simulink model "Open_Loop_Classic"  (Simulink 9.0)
settings: Solver=ode45  StartTime=0.0  StopTime=40  RelTol=1e-3  EnableMultiTasking=on
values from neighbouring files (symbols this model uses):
  d2r = 1/r2d    (= 0.0174532925199)    [init.m]    (also in freq.m; frequ.m; init_lat.m; pl.m)
  r2d = 180/pi    (= 57.2957795131)    [init.m]    (also in freq.m; frequ.m; init_lat.m; pl.m)
undefined symbols (not defined in the file or in its folder): Av, Bv, Cv, Dv

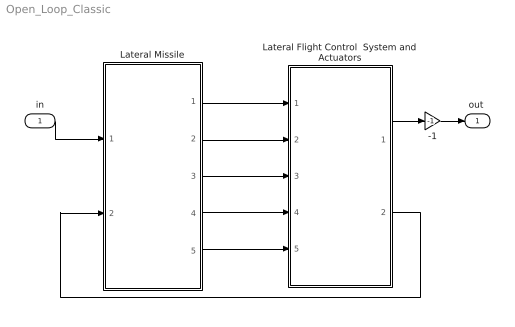
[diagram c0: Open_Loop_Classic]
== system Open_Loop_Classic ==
  in : Inport
  -1 : Gain  Gain=-1
  Lateral Flight Control  System and Actuators : Subsystem
  Lateral Missile : Subsystem
  "out " : Outport
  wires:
  Lateral Missile/1(p) -> Lateral Flight Control  System and Actuators/1(p)
  Lateral Missile/2(phi) -> Lateral Flight Control  System and Actuators/2(phi)
  Lateral Missile/3(r) -> Lateral Flight Control  System and Actuators/3(r)
  Lateral Missile/4(psi) -> Lateral Flight Control  System and Actuators/4(psi)
  Lateral Missile/5(Ny) -> Lateral Flight Control  System and Actuators/5(Nym)
  -1/1 -> "out "/1
  Lateral Flight Control  System and Actuators/1(d-ailer) -> -1/1
  in/1 -> Lateral Missile/1(dail)
  Lateral Flight Control  System and Actuators/2(d-ruddr) -> Lateral Missile/2(drud)

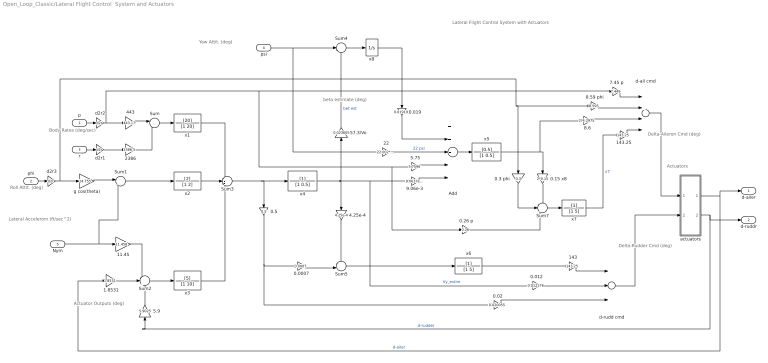
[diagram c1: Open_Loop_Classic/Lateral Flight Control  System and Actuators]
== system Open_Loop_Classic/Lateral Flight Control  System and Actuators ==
  note: Body Rates (deg/sec)
  note: Delta-Rudder Cmd (deg)
  note: Delta-Aileron Cmd (deg)
  note: Lateral Accelerom (ft/sec^2)
  note: Actuator Outputs (deg)
  note: Roll Attit. (deg)
  note: Yaw Attit. (deg)
  note: beta estimate (deg)
  note: Actuators
  note: Lateral Flight Control System with Actuators
  p : Inport
  phi : Inport  Port=2
  r : Inport  Port=3
  psi : Inport  Port=4
  Nym : Inport  Port=5
  0.0007 : Gain  Gain=0.0007
  0.012 : Gain  Gain=0.012176
  0.019 : Gain  Gain=0.019199
  0.02 : Gain  Gain=0.020055
  0.15 x8 : Gain  Gain=2*0.15
  0.26 p : Gain  Gain=0.26
  0.3 phi : Gain  Gain=0.3
  0.5 : Gain  Gain=0.5
  1.8531 : Gain  Gain=1.8531
  11.45 : Gain  Gain=11.458
  143 : Gain  Gain=143.25
  143.25 : Gain  Gain=143.25
  22 : Gain  Gain=22.002*d2r
  2386 : Gain  Gain=2386.5
  4.25e-4 : Gain  Gain=4.25e-4
  443 : Gain  Gain=443.17
  5.75 : Gain  Gain=5.7596
  5.9 : Gain  Gain=5.9025
  57.3/Vo : Gain  Gain=0.023605
  7.45 p : Gain  Gain=7.449
  8.59 phi : Gain  Gain=8.595
  8.6 : Gain  Gain=2*4.2975
  "9.06e-3 " : Gain  Gain=9.0637e-3
  Add : Sum  Inputs=++---
  Sum : Sum  Inputs=|-+
  Sum1 : Sum  Inputs=|++
  Sum2 : Sum  Inputs=-++
  Sum3 : Sum  Inputs=-++
  Sum4 : Sum  Inputs=+--
  Sum5 : Sum  Inputs=--|
  Sum7 : Sum  Inputs=-++
  actuators : Subsystem
  d-ail cmd : Sum  Inputs=++-+
  d-rudd cmd : Sum  Inputs=+--
  d2r1 : Gain  Gain=d2r
  d2r2 : Gain  Gain=d2r
  d2r3 : Gain  Gain=d2r
  g cos(theta) : Gain  Gain=24.755
  x1 : TransferFcn  Numerator=[20]  Denominator=[1 20]
  x2 : TransferFcn  Numerator=[2]  Denominator=[1 2]
  x3 : TransferFcn  Numerator=[5]  Denominator=[1 10]
  x4 : TransferFcn  Denominator=[1 0.5]
  x5 : TransferFcn  Numerator=[0.5]  Denominator=[1 0.5]
  x6 : TransferFcn  Denominator=[1 5]
  x7 : TransferFcn  Denominator=[1 5]
  x8 : Integrator
  d-ailer : Outport
  d-ruddr : Outport  Port=2
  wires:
  0.5/1 -> 0.02/1, 0.0007/1
  d-rudd cmd/1 -> actuators/2(dr)
  0.02/1 -> d-rudd cmd/3
  0.012/1 -> d-rudd cmd/2
  x6/1 -> 143/1
  143/1 -> d-rudd cmd/1
  d-ail cmd/1 -> actuators/1(da)
  7.45 p/1 -> d-ail cmd/1
  8.59 phi/1 -> d-ail cmd/2
  143.25/1 -> d-ail cmd/4
  x7/1 -> 143.25/1  "x7"
  8.6/1 -> d-ail cmd/3
  0.3 phi/1 -> Sum7/2
  0.26 p/1 -> Sum7/3
  0.15 x8/1 -> Sum7/1
  Sum7/1 -> x7/1
  x5/1 -> 8.6/1, 0.15 x8/1
  5.75/1 -> Add/4
  22/1 -> Add/3  "22 psi"
  0.019/1 -> Add/2
  x8/1 -> 0.019/1
  Add/1 -> x5/1
  "9.06e-3 "/1 -> Add/5
  Sum5/1 -> x6/1
  0.0007/1 -> Sum5/2
  4.25e-4/1 -> Sum5/1
  Nym/1 -> Sum1/2, 11.45/1
  Sum4/1 -> x8/1
  57.3/Vo/1 -> Sum4/3  "bet est"
  x4/1 -> 0.012/1, "9.06e-3 "/1, 4.25e-4/1, 57.3/Vo/1  "Vy_estim"
  psi/1 -> Sum4/2, 22/1
  Sum3/1 -> 0.5/1, x4/1
  x3/1 -> Sum3/3
  x2/1 -> Sum3/2
  x1/1 -> Sum3/1
  Sum2/1 -> x3/1
  5.9/1 -> Sum2/3
  1.8531/1 -> Sum2/2
  11.45/1 -> Sum2/1
  phi/1 -> d2r3/1
  g cos(theta)/1 -> Sum1/1
  Sum1/1 -> x2/1
  2386/1 -> Sum/2
  r/1 -> d2r1/1
  p/1 -> d2r2/1
  443/1 -> Sum/1
  Sum/1 -> x1/1
  actuators/1("da ") -> d-ailer/1, 1.8531/1  "d-ailer"
  actuators/2("dr ") -> d-ruddr/1, 5.9/1  "d-rudder"
  d2r3/1 -> 8.59 phi/1, 0.3 phi/1, g cos(theta)/1
  d2r2/1 -> 7.45 p/1, 0.26 p/1, 5.75/1, 443/1
  d2r1/1 -> 2386/1

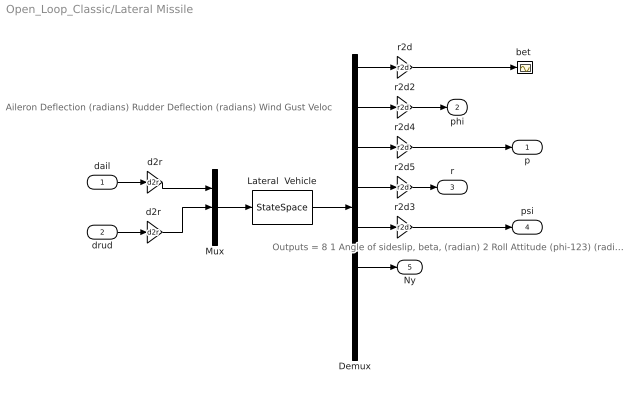
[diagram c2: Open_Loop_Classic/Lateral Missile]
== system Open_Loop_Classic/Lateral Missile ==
  note: Aileron Deflection (radians) Rudder Deflection (radians) Wind Gust Veloc
  note: Outputs = 8 1 Angle of sideslip, beta, (radian) 2 Roll Attitude (phi-123) (radians) 3 Roll Rate (p-body) (rad/sec) 4 Yaw Rate (r-body) (rad/sec) 5 Yaw Attitude (psi-123) (radians) 6 Y-Acceleromet, (ft/sec^2) Translation 7 Cross Range Velocity (Vcr) (ft/sec) 8 Beta Sensed at Vane # 1 (radian)
  dail : Inport
  drud : Inport  Port=2
  Demux : Demux  Outputs=8
  Lateral  Vehicle : StateSpace  A=Av  B=Bv  C=Cv  D=Dv  InitialCondition=0
  Mux : Mux  Inputs=3
  "bet " : Scope
  d2r : Gain  Gain=d2r
  "d2r " : Gain  Gain=d2r
  r2d{,2..5} (5 alike) : Gain  Gain=r2d
  p : Outport
  phi : Outport  Port=2
  r : Outport  Port=3
  psi : Outport  Port=4
  Ny : Outport  Port=5
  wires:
  Mux/1 -> Lateral  Vehicle/1
  Lateral  Vehicle/1 -> Demux/1
  dail/1 -> d2r/1
  drud/1 -> "d2r "/1
  r2d/1 -> "bet "/1
  Demux/1 -> r2d/1
  Demux/2 -> r2d2/1
  Demux/3 -> r2d4/1
  Demux/4 -> r2d5/1
  Demux/5 -> r2d3/1
  Demux/6 -> Ny/1
  r2d2/1 -> phi/1
  r2d3/1 -> psi/1
  r2d4/1 -> p/1
  r2d5/1 -> r/1
  d2r/1 -> Mux/1
  "d2r "/1 -> Mux/2

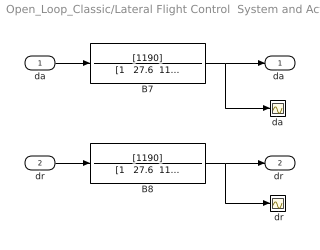
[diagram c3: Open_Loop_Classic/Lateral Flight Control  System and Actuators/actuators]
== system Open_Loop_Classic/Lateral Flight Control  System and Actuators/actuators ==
  da : Inport
  dr : Inport  Port=2
  " da " : Scope
  " dr" : Scope
  B7 : TransferFcn  Numerator=[1190]  Denominator="[1   27.6  1190]"
  B8 : TransferFcn  Numerator=[1190]  Denominator="[1   27.6  1190]"
  "da " : Outport
  "dr " : Outport  Port=2
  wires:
  B8/1 -> " dr"/1, "dr "/1
  dr/1 -> B8/1
  B7/1 -> " da "/1, "da "/1
  da/1 -> B7/1
